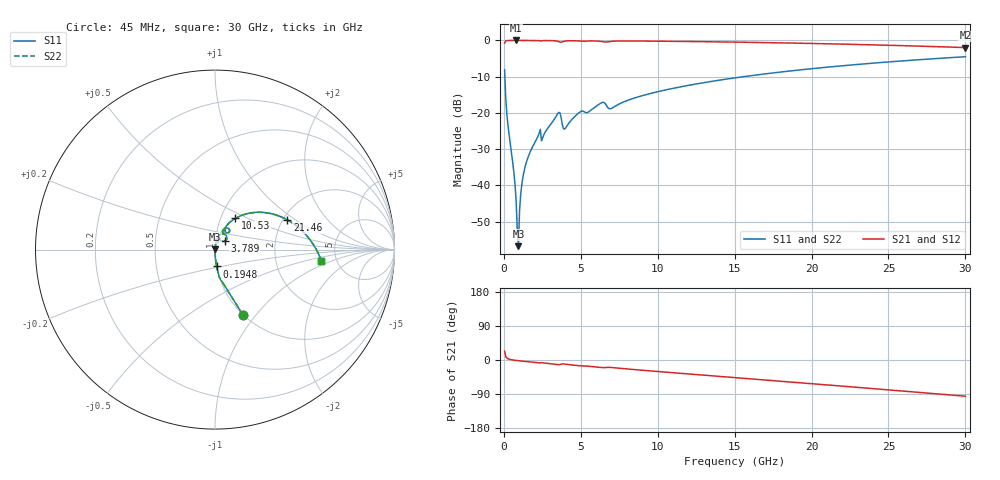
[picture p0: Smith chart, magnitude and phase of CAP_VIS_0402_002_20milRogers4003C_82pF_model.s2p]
! S-parameter model data by Modelithics Inc.  support@modelithics.com  813-866-6335  Tampa FL USA
! S-Parameter data specifications:
! Substrate: 20-mil Rogers 4003C, substrate thickness, H=0.508mm, Dielectric constant, Er=3.75
! PCB Mounting Pad Footprint: Pad width, PadW=0.50mm , Pad length, PadL=0.50mm , Pad gap, PadG (edge-to-edge)=0.40mm , Reference planes=1.4mm apart
! Created Wed Nov 18 12:57:12 2015
# hz S ma R 50
! 2 Port Network Data from SP1.SP block
! freq  magS11  angS11  magS21  angS21  magS12  angS12  magS22  angS22
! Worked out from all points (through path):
!   401 points, 45 MHz to 30 GHz, reference 50 ohm
!   highest |S21| = -0.01 dB at 793.9 MHz (marker M1); lowest = -2.0 dB at 30 GHz (marker M2)
!   group delay of S21, straight-line fit = 8.95 ps
!   lowest |S11| = -56.8 dB at 943.6 MHz (marker M3), VSWR 1.00, Z = 50.1 + j0.12 ohm
!   |S11| at or under -10 dB: 62.77 MHz to 15.59 GHz (15.52 GHz wide, 198 % of centre)
!   |S22| runs from -56.8 to -4.5 dB; largest |S21 - S12| = 0
!   S11 on the Smith chart (normalised r, x): 45 MHz: 1.00, -0.86; 194.8 MHz: 1.00, -0.19; 3.789 GHz: 1.11, +0.10; 10.53 GHz: 1.17, +0.43; 21.46 GHz: 2.12, +0.86; 30 GHz: 3.80, -0.74
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4.5e7  0.3936 -66.9  0.9191 23.1  0.9191 23.1  0.3936 -66.9
1.94775e8  0.09429 -84.7  0.9952 5.0  0.9952 5.0  0.09429 -84.7
6.441e8  0.01526 -87.9  0.9992 -0.4  0.9992 -0.4  0.01526 -87.9
7.93875e8  0.006168 -84.5  0.9992 -1.2  0.9992 -1.2  0.006168 -84.5
9.4365e8  0.001445 55.7  0.9992 -1.9  0.9992 -1.9  0.001445 55.7
1.018538e9  0.00455 77.6  0.9992 -2.2  0.9992 -2.2  0.00455 77.6
1.168312e9  0.01048 82.4  0.999 -2.8  0.999 -2.8  0.01048 82.4
1.318088e9  0.01594 83.3  0.9989 -3.4  0.9989 -3.4  0.01594 83.3
1.767412e9  0.03092 82.7  0.9983 -5.1  0.9983 -5.1  0.03092 82.7
2.216738e9  0.04762 80.3  0.9965 -7.0  0.9965 -7.0  0.04762 80.3
2.591175e9  0.04984 78.9  0.9958 -7.8  0.9958 -7.8  0.04984 78.9
3.489825e9  0.09696 65.9  0.9753 -12.1  0.9753 -12.1  0.09696 65.9
3.789375e9  0.07036 41.1  0.9545 -10.4  0.9545 -10.4  0.07036 41.1
4.014038e9  0.06198 63.5  0.9816 -11.1  0.9816 -11.1  0.06198 63.5
5.062462e9  0.106 65.7  0.9785 -15.7  0.9785 -15.7  0.106 65.7
1.007992e10  0.1977 58.3  0.9762 -30.6  0.9762 -30.6  0.1977 58.3
1.052925e10  0.2078 56.9  0.9742 -32.1  0.9742 -32.1  0.2078 56.9
1.50225e10  0.3044 42.9  0.9484 -46.4  0.9484 -46.4  0.3044 42.9
2.003996e10  0.4079 26.9  0.9084 -62.6  0.9084 -62.6  0.4079 26.9
2.146282e10  0.4364 22.3  0.8949 -67.2  0.8949 -67.2  0.4364 22.3
2.505742e10  0.5062 10.5  0.8572 -79.0  0.8572 -79.0  0.5062 10.5
3e10  0.5962 -6.0  0.7968 -95.6  0.7968 -95.6  0.5962 -6.0
